| TEXAS INSTRUMENTS INCORPORATED
| Standard Linear and Logic Group
| IBIS Model of SN74AHC574
| OCTAL EDGE-TRIGGERED D-TYPE FLIP-FLOPS WITH 3-STATE OUTPUTS
| This file contains package information for the following:
|  SSOP 20-pin (DB) package as [Component] AHC574_DB
|  TVSOP 20-pin (DGV) package as [Component] AHC574_DGV
|  SOIC 20-pin (DW) package as [Component] AHC574_DW
|  PDIP 20-pin (N) package as [Component] AHC574_N
|  SOP 20-pin (NS) package as [Component] AHC574_NS
|  TSSOP 20-pin (PW) package as [Component] AHC574_PW
| This device can be powered at the following Vccs:
|  2.2 volt Vcc
|  3.3 volt Vcc
|  5 volt Vcc
| This file provides unique models under the [Model Selector] for each Vcc.
| For operation at a specific Vcc, select the appropriate model after each
| [Model Selector] keyword.
[IBIS Ver]   3.2
[Comment char]  |_char
[File Name]   sn74ahc574.ibs
[File Rev]   1.1 | a_die
[Date]   November 27, 2002
[Source]   Data created from TI-SPICE simulations at TI-SLL.
[Notes]   The following is an IBIS list for the AHC574.
   Please contact sllibis@ti.com with questions and
   comments concerning SLL IBIS models.
   This IBIS model is created from a BA (back annotated
   netlist).
   -Due to the fact that the Device is 5-V Input/Output
   tolarent, the output model has some Non-Monotonic Warnings.
   -Power-clamp data has been deleted from the OE and CLK models
   since there is no power-clamp diode.
[Disclaimer] Property of Texas Instruments Incorporated.  Unauthorized
   reproduction and/or distribution is strictly prohibited.
   This product is protected under copyright law.
   Created  2002, (C) Copyright  2002, Texas Instruments
   Incorporated, All Rights Reserved
   UNLESS THERE IS A SIGNED, WRITTEN AGREEMENT TO THE
   CONTRARY, TEXAS INSTRUMENTS (TI) IS PROVIDING THE IBIS
   MODELS  AND WITHOUT ANY WARRANTY, EXPRESSED OR
   IMPLIED.  TI assumes no liability for:
   1) the accuracy of the IBIS models provided to your
   company;
   2) the proper functioning of these IBIS Models in your
   design or for any resulting applications; or
   3) infringement of patents, copyrights or intellectual
   property rights resulting from your use of these IBIS
   models.
   TI provides IBIS Models as a service to our customers.
   You and your company shall not distribute, sell or give
   these models to anyone else without prior written
   permission from TI.
   TI reserves the right to make changes to our products or
   to discontinue any semiconductor product or service
   without notice, and advises our customers to obtain the
   latest version of relevant information to verify, before
   placing orders, that the information being relied on is
   current.
   Please be aware that your receipt and use of the IBIS
   information provided shall serve as acceptance of these
   terms and conditions.  If you do not accept these terms,
   you should return or destroy the IBIS models and any
   other accompanying information immediately.
| Component AHC574_DB 20-pin SSOP
[Component]   AHC574_DB
[Manufacturer]   Texas Instruments, Inc.
[Package]
|   typ   min   max
R_pkg   4.000e-02   3.500e-02   5.100e-02
L_pkg   3.495e-09   3.035e-09   4.314e-09
C_pkg   4.200e-13   3.460e-13   5.020e-13
[Pin]   signal_name   model_name   R_pin   L_pin   C_pin
1   NOE   AHC574_OE   4.900e-02   4.310e-09   5.020e-13
2   1D   AHC574_IN   4.800e-02   3.903e-09   4.870e-13
3   2D   AHC574_IN   3.500e-02   3.189e-09   3.960e-13
4   3D   AHC574_IN   3.500e-02   3.036e-09   3.470e-13
5   4D   AHC574_IN   3.500e-02   3.035e-09   3.670e-13
6   5D   AHC574_IN   3.500e-02   3.035e-09   3.670e-13
7   6D   AHC574_IN   3.500e-02   3.036e-09   3.470e-13
8   7D   AHC574_IN   3.500e-02   3.189e-09   3.970e-13
9   8D   AHC574_IN   4.700e-02   3.899e-09   4.880e-13
10   GND   GND   5.100e-02   4.314e-09   5.000e-13
11   CLK   AHC574_CLK   5.100e-02   4.314e-09   5.000e-13
12   8Q   AHC574_OUT   4.700e-02   3.899e-09   4.880e-13
13   7Q   AHC574_OUT   3.500e-02   3.189e-09   3.970e-13
14   6Q   AHC574_OUT   3.500e-02   3.036e-09   3.460e-13
15   5Q   AHC574_OUT   3.500e-02   3.035e-09   3.670e-13
16   4Q   AHC574_OUT   3.500e-02   3.035e-09   3.670e-13
17   3Q   AHC574_OUT   3.500e-02   3.036e-09   3.460e-13
18   2Q   AHC574_OUT   3.500e-02   3.189e-09   3.970e-13
19   1Q   AHC574_OUT   4.700e-02   3.899e-09   4.880e-13
20   VCC   POWER   5.100e-02   4.314e-09   5.020e-13
| Component AHC574_DGV 20-pin TVSOP
[Component]   AHC574_DGV
[Manufacturer]   Texas Instruments, Inc.
[Package]
|   typ   min   max
R_pkg   4.400e-02   3.800e-02   4.800e-02
L_pkg   2.561e-09   2.236e-09   2.961e-09
C_pkg   3.420e-13   2.640e-13   4.460e-13
[Pin]   signal_name   model_name   R_pin   L_pin   C_pin
1   NOE   AHC574_OE   4.400e-02   2.935e-09   4.170e-13
2   1D   AHC574_IN   4.200e-02   2.869e-09   4.460e-13
3   2D   AHC574_IN   4.300e-02   2.399e-09   3.160e-13
4   3D   AHC574_IN   4.400e-02   2.236e-09   2.650e-13
5   4D   AHC574_IN   4.600e-02   2.278e-09   2.640e-13
6   5D   AHC574_IN   4.500e-02   2.274e-09   2.640e-13
7   6D   AHC574_IN   4.400e-02   2.285e-09   2.690e-13
8   7D   AHC574_IN   4.300e-02   2.452e-09   3.200e-13
9   8D   AHC574_IN   4.400e-02   2.900e-09   4.460e-13
10   GND   GND   4.400e-02   2.961e-09   4.180e-13
11   CLK   AHC574_CLK   4.500e-02   2.954e-09   4.180e-13
12   8Q   AHC574_OUT   4.200e-02   2.847e-09   4.430e-13
13   7Q   AHC574_OUT   4.500e-02   2.453e-09   3.190e-13
14   6Q   AHC574_OUT   4.500e-02   2.297e-09   2.690e-13
15   5Q   AHC574_OUT   4.800e-02   2.334e-09   2.680e-13
16   4Q   AHC574_OUT   4.800e-02   2.335e-09   2.670e-13
17   3Q   AHC574_OUT   4.600e-02   2.299e-09   2.680e-13
18   2Q   AHC574_OUT   4.600e-02   2.457e-09   3.200e-13
19   1Q   AHC574_OUT   4.300e-02   2.848e-09   4.410e-13
20   VCC   POWER   3.800e-02   2.812e-09   4.080e-13
| Component AHC574_DW 20-pin SOIC
[Component]   AHC574_DW
[Manufacturer]   Texas Instruments, Inc.
[Package]
|   typ   min   max
R_pkg   3.800e-02   3.300e-02   4.500e-02
L_pkg   5.012e-09   4.110e-09   6.349e-09
C_pkg   7.170e-13   5.300e-13   8.680e-13
[Pin]   signal_name   model_name   R_pin   L_pin   C_pin
1   NOE   AHC574_OE   4.200e-02   6.336e-09   8.650e-13
2   1D   AHC574_IN   4.300e-02   5.542e-09   8.670e-13
3   2D   AHC574_IN   3.400e-02   4.714e-09   7.320e-13
4   3D   AHC574_IN   3.400e-02   4.377e-09   5.910e-13
5   4D   AHC574_IN   3.600e-02   4.130e-09   5.330e-13
6   5D   AHC574_IN   3.500e-02   4.111e-09   5.300e-13
7   6D   AHC574_IN   3.400e-02   4.284e-09   5.830e-13
8   7D   AHC574_IN   3.400e-02   4.634e-09   7.260e-13
9   8D   AHC574_IN   4.000e-02   5.518e-09   8.650e-13
10   GND   GND   4.300e-02   6.349e-09   8.660e-13
11   CLK   AHC574_CLK   4.100e-02   6.281e-09   8.610e-13
12   8Q   AHC574_OUT   4.500e-02   5.561e-09   8.680e-13
13   7Q   AHC574_OUT   3.300e-02   4.778e-09   7.420e-13
14   6Q   AHC574_OUT   3.500e-02   4.414e-09   5.960e-13
15   5Q   AHC574_OUT   3.500e-02   4.110e-09   5.330e-13
16   4Q   AHC574_OUT   3.600e-02   4.130e-09   5.330e-13
17   3Q   AHC574_OUT   3.400e-02   4.377e-09   5.910e-13
18   2Q   AHC574_OUT   3.400e-02   4.714e-09   7.310e-13
19   1Q   AHC574_OUT   4.300e-02   5.569e-09   8.680e-13
20   VCC   POWER   4.200e-02   6.308e-09   8.640e-13
| Component AHC574_N 20-pin PDIP
[Component]   AHC574_N
[Manufacturer]   Texas Instruments, Inc.
[Package]
|   typ   min   max
R_pkg   4.300e-02   3.800e-02   5.000e-02
L_pkg   7.384e-09   4.680e-09   1.032e-08
C_pkg   5.100e-13   2.310e-13   8.210e-13
[Pin]   signal_name   model_name   R_pin   L_pin   C_pin
1   NOE   AHC574_OE   4.200e-02   9.427e-09   8.100e-13
2   1D   AHC574_IN   4.600e-02   8.544e-09   4.560e-13
3   2D   AHC574_IN   4.800e-02   7.163e-09   4.350e-13
4   3D   AHC574_IN   4.000e-02   4.825e-09   2.610e-13
5   4D   AHC574_IN   4.000e-02   5.284e-09   6.480e-13
6   5D   AHC574_IN   4.000e-02   4.686e-09   2.320e-13
7   6D   AHC574_IN   4.000e-02   6.359e-09   4.890e-13
8   7D   AHC574_IN   3.800e-02   7.982e-09   4.750e-13
9   8D   AHC574_IN   4.300e-02   9.403e-09   4.750e-13
10   GND   GND   5.000e-02   1.032e-08   8.050e-13
11   CLK   AHC574_CLK   5.000e-02   1.028e-08   8.100e-13
12   8Q   AHC574_OUT   4.300e-02   9.383e-09   4.770e-13
13   7Q   AHC574_OUT   3.800e-02   7.978e-09   4.760e-13
14   6Q   AHC574_OUT   4.000e-02   6.302e-09   4.920e-13
15   5Q   AHC574_OUT   4.000e-02   4.680e-09   2.310e-13
16   4Q   AHC574_OUT   4.000e-02   5.284e-09   6.480e-13
17   3Q   AHC574_OUT   4.000e-02   4.822e-09   2.610e-13
18   2Q   AHC574_OUT   4.700e-02   7.118e-09   4.390e-13
19   1Q   AHC574_OUT   4.600e-02   8.492e-09   4.610e-13
20   VCC   POWER   4.300e-02   9.348e-09   8.210e-13
| Component AHC574_NS 20-pin SOP
[Component]   AHC574_NS
[Manufacturer]   Texas Instruments, Inc.
[Package]
|   typ   min   max
R_pkg   4.400e-02   2.900e-02   5.800e-02
L_pkg   3.666e-09   2.317e-09   5.115e-09
C_pkg   5.480e-13   3.160e-13   7.250e-13
[Pin]   signal_name   model_name   R_pin   L_pin   C_pin
1   NOE   AHC574_OE   5.800e-02   5.115e-09   7.250e-13
2   1D   AHC574_IN   5.300e-02   4.591e-09   7.240e-13
3   2D   AHC574_IN   4.900e-02   3.754e-09   5.720e-13
4   3D   AHC574_IN   2.900e-02   2.549e-09   3.880e-13
5   4D   AHC574_IN   3.100e-02   2.317e-09   3.160e-13
6   5D   AHC574_IN   3.100e-02   2.317e-09   3.160e-13
7   6D   AHC574_IN   2.900e-02   2.556e-09   3.990e-13
8   7D   AHC574_IN   4.900e-02   3.754e-09   5.790e-13
9   8D   AHC574_IN   5.300e-02   4.591e-09   7.240e-13
10   GND   GND   5.800e-02   5.115e-09   7.250e-13
11   CLK   AHC574_CLK   5.800e-02   5.115e-09   7.250e-13
12   8Q   AHC574_OUT   5.300e-02   4.591e-09   7.240e-13
13   7Q   AHC574_OUT   4.900e-02   3.754e-09   5.790e-13
14   6Q   AHC574_OUT   2.900e-02   2.557e-09   3.990e-13
15   5Q   AHC574_OUT   3.100e-02   2.317e-09   3.160e-13
16   4Q   AHC574_OUT   3.100e-02   2.317e-09   3.160e-13
17   3Q   AHC574_OUT   2.900e-02   2.557e-09   3.990e-13
18   2Q   AHC574_OUT   4.900e-02   3.754e-09   5.790e-13
19   1Q   AHC574_OUT   5.300e-02   4.591e-09   7.240e-13
20   VCC   POWER   5.800e-02   5.115e-09   7.250e-13
| Component AHC574_PW 20-pin TSSOP
[Component]   AHC574_PW
[Manufacturer]   Texas Instruments, Inc.
[Package]
|   typ   min   max
R_pkg   5.000e-02   4.200e-02   6.000e-02
L_pkg   2.802e-09   2.248e-09   3.553e-09
C_pkg   3.170e-13   2.020e-13   4.430e-13
[Pin]   signal_name   model_name   R_pin   L_pin   C_pin
1   NOE   AHC574_OE   5.500e-02   3.461e-09   4.400e-13
2   1D   AHC574_IN   5.500e-02   3.150e-09   4.010e-13
3   2D   AHC574_IN   4.200e-02   2.619e-09   3.020e-13
4   3D   AHC574_IN   4.500e-02   2.273e-09   2.020e-13
5   4D   AHC574_IN   4.500e-02   2.248e-09   2.240e-13
6   5D   AHC574_IN   4.500e-02   2.273e-09   2.260e-13
7   6D   AHC574_IN   4.400e-02   2.323e-09   2.050e-13
8   7D   AHC574_IN   4.600e-02   2.704e-09   3.070e-13
9   8D   AHC574_IN   6.000e-02   3.265e-09   4.110e-13
10   GND   GND   5.700e-02   3.506e-09   4.360e-13
11   CLK   AHC574_CLK   5.800e-02   3.553e-09   4.370e-13
12   8Q   AHC574_OUT   5.800e-02   3.193e-09   4.050e-13
13   7Q   AHC574_OUT   4.200e-02   2.704e-09   3.110e-13
14   6Q   AHC574_OUT   4.600e-02   2.392e-09   2.100e-13
15   5Q   AHC574_OUT   4.700e-02   2.334e-09   2.290e-13
16   4Q   AHC574_OUT   4.700e-02   2.300e-09   2.270e-13
17   3Q   AHC574_OUT   4.700e-02   2.349e-09   2.070e-13
18   2Q   AHC574_OUT   4.500e-02   2.677e-09   3.060e-13
19   1Q   AHC574_OUT   6.000e-02   3.235e-09   4.060e-13
20   VCC   POWER   5.600e-02   3.487e-09   4.430e-13
| Model AHC574_CLK
[Model Selector]   AHC574_CLK
AHC574_CLK_22   2.2 volt Vcc
AHC574_CLK_33   3.3 volt Vcc
AHC574_CLK_50   5 volt Vcc
| Model AHC574_OE
[Model Selector]   AHC574_OE
AHC574_OE_22   2.2 volt Vcc
AHC574_OE_33   3.3 volt Vcc
AHC574_OE_50   5 volt Vcc
| Model AHC574_IN
[Model Selector]   AHC574_IN
AHC574_IN_22   2.2 volt Vcc
AHC574_IN_33   3.3 volt Vcc
AHC574_IN_50   5 volt Vcc
| Model AHC574_OUT
[Model Selector]   AHC574_OUT
AHC574_OUT_22   2.2 volt Vcc
AHC574_OUT_33   3.3 volt Vcc
AHC574_OUT_50   5 volt Vcc
| Models and submodels in the file (12): AHC574_CLK_22 (Input), AHC574_CLK_33 (Input), AHC574_CLK_50 (Input), AHC574_OE_22 (Input), AHC574_OE_33 (Input), AHC574_OE_50 (Input), AHC574_IN_22 (Input), AHC574_IN_33 (Input), AHC574_IN_50 (Input), AHC574_OUT_22 (3-state), AHC574_OUT_33 (3-state), AHC574_OUT_50 (3-state)
